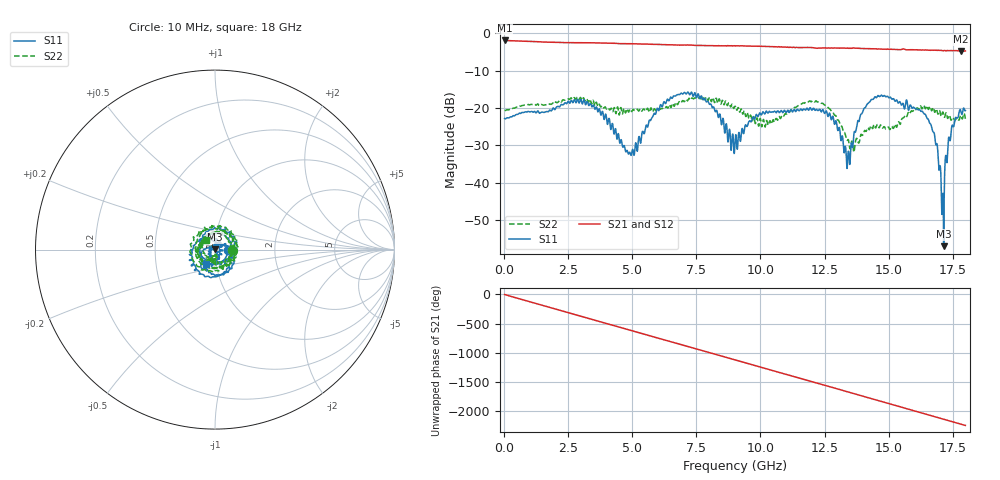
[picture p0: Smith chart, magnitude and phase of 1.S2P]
!Agilent Technologies,E5071C,MY46316741,A.11.02
!Date: Fri May 06 15:18:45 2022
!Data & Calibration Information:
!Freq	S11:SOLT2(ON)	S21:SOLT2(ON)	S12:SOLT2(ON)	S22:SOLT2(ON)
!PortZ  Port1:50+j0  Port2:50+j0
!Above PortZ is port z conversion or system Z0 setting when saving the data.
!When reading, reference impedance value at option line is always used.
# Hz S dB R 50
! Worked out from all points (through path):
!   1800 points, 10 MHz to 18 GHz, reference 50 ohm
!   highest |S21| = -1.94 dB at 10 MHz (marker M1); lowest = -4.8 dB at 17.84 GHz (marker M2)
!   group delay of S21, straight-line fit = 347 ps
!   lowest |S11| = -57.0 dB at 17.15 GHz (marker M3), VSWR 1.00, Z = 50 + j0.139 ohm
!   |S11| at or under -10 dB: start of sweep to end of sweep
!   |S22| runs from -31.8 to -17.0 dB; largest |S21 - S12| = 0.049
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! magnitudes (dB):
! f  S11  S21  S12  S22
! 10 MHz  -22.8  -1.9  -2.0  -20.6
! 3.01 GHz  -18.2  -2.5  -2.6  -17.7
! 3.9 GHz  -23.1  -2.6  -2.6  -19.9
! 4.89 GHz  -31.9  -2.8  -2.8  -20.5
! 6.01 GHz  -20.6  -3.0  -3.0  -20.3
! 6.83 GHz  -16.4  -3.2  -3.2  -18.3
! 7.63 GHz  -17.6  -3.3  -3.3  -17.1
! 9.01 GHz  -28.6  -3.4  -3.4  -19.5
! 10.24 GHz  -20.9  -3.6  -3.6  -23.4
! 12.01 GHz  -20.6  -3.8  -3.9  -18.2
! 12.89 GHz  -24.4  -4.0  -4.0  -22.0
! 13.43 GHz  -31.6  -4.0  -4.0  -28.5
! 14.1 GHz  -19.8  -4.1  -4.2  -26.2
! 15.01 GHz  -17.3  -4.3  -4.3  -25.2
! 16.5 GHz  -22.7  -4.5  -4.6  -19.4
! 16.83 GHz  -29.3  -4.6  -4.6  -20.8
! 17.08 GHz  -48.5  -4.6  -4.7  -21.8
! 17.15 GHz  -57.0  -4.7  -4.7  -21.8
! 17.28 GHz  -34.7  -4.6  -4.7  -22.1
! 17.41 GHz  -28.7  -4.7  -4.8  -22.6
! 17.84 GHz  -21.4  -4.8  -4.9  -22.2
! 18 GHz  -20.7  -4.8  -4.9  -22.9
